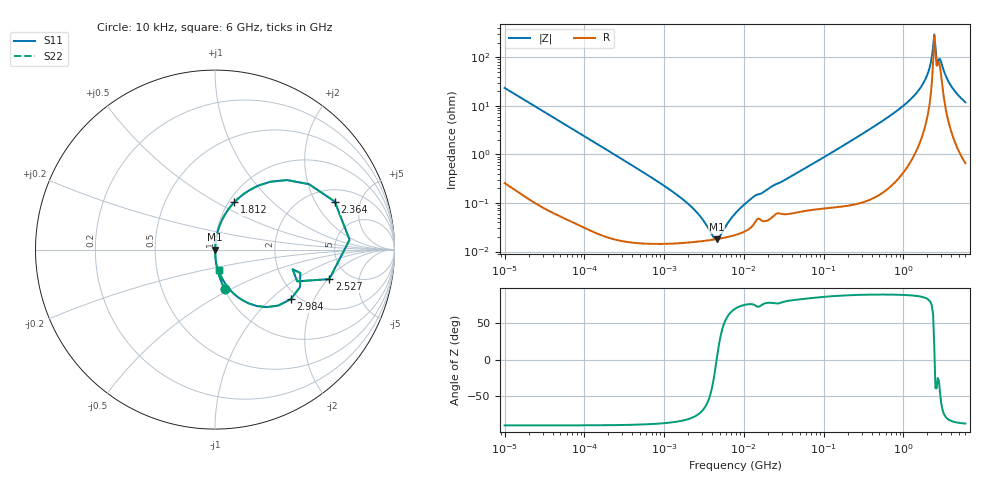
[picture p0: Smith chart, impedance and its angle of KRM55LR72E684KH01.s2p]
!Murata Part Number: KRM55LR72E684KH01
!These Parameters are Measured in Series Mode Connection
!Data Generated on Jan 08, 2026
!  o--ll--o
!Port1  Port2
!  o------o
!Operation Temp=25[degC], DC Bias Voltage=0[V]
!Freq. Start=10[kHz] Stop=6[GHz] 401[Steps]
# Hz S RI R 50
!Freq.(Hz) S11(Real) S11(Imag) S21(Real) S21(Imag) S12(Real) S12(Imag) S22(Real) S22(Imag)
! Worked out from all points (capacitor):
!   401 points, 10 kHz to 6 GHz, reference 50 ohm
!   read as one part in series: C = 680 nF near 10.69 kHz
!   lowest |Z| = 18 mohm at 4.549 MHz (marker M1)
!   series resonance near 4.562 MHz, so ESL is about 1.8 nH
!   S11 on the Smith chart (normalised r, x): 10 kHz: 1.01, -0.47; 1.812 GHz: 1.06, +0.61; 2.364 GHz: 2.65, +2.94; 2.527 GHz: 3.57, -2.07; 2.984 GHz: 1.81, -1.35; 6 GHz: 1.01, -0.24
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10000  0.0539 -0.2204  0.9461 0.2204  0.9461 0.2204  0.0539 -0.2204
26237  0.00884 -0.0887  0.9912 0.0887  0.9912 0.0887  0.00884 -0.0887
92862  0.000973 -0.0254  0.999 0.0254  0.999 0.0254  0.000973 -0.0254
862344  0.000151 -0.00265  0.9998 0.00265  0.9998 0.00265  0.000151 -0.00265
2262542  0.000157 -0.000782  0.9998 0.000782  0.9998 0.000782  0.000157 -0.000782
3052144  0.000165 -0.000423  0.9998 0.000423  0.9998 0.000423  0.000165 -0.000423
4117309  0.000176 -0.000105  0.9998 0.000105  0.9998 0.000105  0.000176 -0.000105
4549352  0.00018 -2.8e-06  0.9998 2.8e-06  0.9998 2.8e-06  0.00018 -2.8e-06
7745967  0.000218 0.00056  0.9998 -0.00056  0.9998 -0.00056  0.000218 0.00056
1.363475e7  0.000388 0.00134  0.9996 -0.00134  0.9996 -0.00134  0.000388 0.00134
7.193098e7  0.000759 0.00625  0.9992 -0.00625  0.9992 -0.00625  0.000759 0.00625
6.67969e8  0.00573 0.0604  0.9943 -0.0604  0.9943 -0.0604  0.00573 0.0604
1.256662e9  0.0262 0.1353  0.9738 -0.1353  0.9738 -0.1353  0.0262 0.1353
1.811831e9  0.1083 0.2645  0.8917 -0.2645  0.8917 -0.2645  0.1083 0.2645
2.139659e9  0.308 0.3779  0.692 -0.3779  0.692 -0.3779  0.308 0.3779
2.286837e9  0.5236 0.3647  0.4764 -0.3647  0.4764 -0.3647  0.5236 0.3647
2.364181e9  0.6673 0.2677  0.3327 -0.2677  0.3327 -0.2677  0.6673 0.2677
2.526803e9  0.6365 -0.1647  0.3635 0.1647  0.3635 0.1647  0.6365 -0.1647
2.983997e9  0.4215 -0.277  0.5785 0.277  0.5785 0.277  0.4215 -0.277
3.297118e9  0.2323 -0.314  0.7677 0.314  0.7677 0.314  0.2323 -0.314
3.766309e9  0.1093 -0.2498  0.8907 0.2498  0.8907 0.2498  0.1093 -0.2498
6e9  0.0199 -0.1147  0.9801 0.1147  0.9801 0.1147  0.0199 -0.1147
